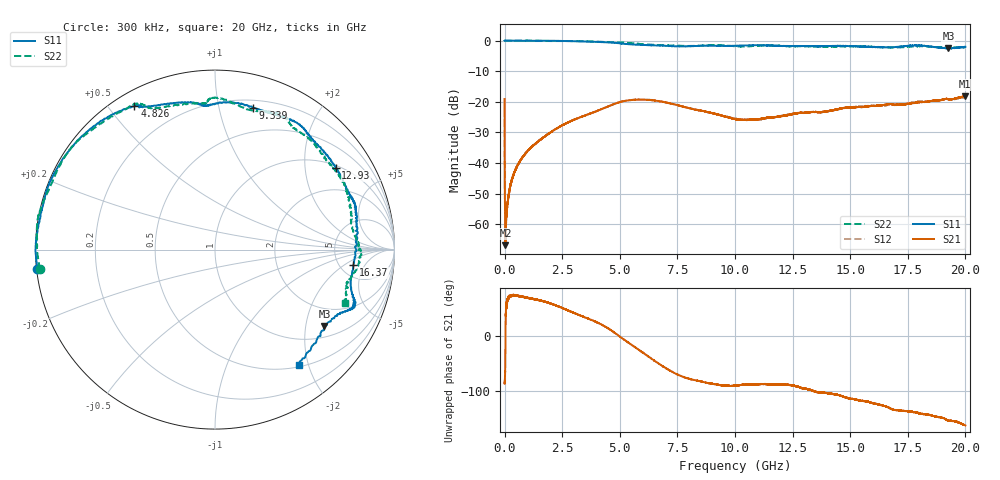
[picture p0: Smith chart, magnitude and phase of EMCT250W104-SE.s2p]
!EMCT250W104
!Johanson Technology Inc.
!www.johansontechnology.com
!Test Board Conditions:
!Substrate Type  RO4350B
!Substrate Thickness  10 mil
!Substrate Dk  3.66
!TL Type: GCPW
!TL Trace Width  22 mil
!TL Gap  14 mil
!PART MODE SINGLE ENDED (AKA BYPASS)
!DUT TOPOLOGY	SERIES-SHUNT
# MHz S  dB  R 50
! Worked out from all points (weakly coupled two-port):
!   20001 points, 300 kHz to 20 GHz, reference 50 ohm
!   highest |S21| = -18.23 dB at 20 GHz (marker M1); lowest = -66.9 dB at 38.3 MHz (marker M2)
!   lowest |S11| = -2.6 dB at 19.26 GHz (marker M3), VSWR 6.80, Z = 67 - j128 ohm
!   |S11| at or under -10 dB: nowhere
!   |S22| runs from -2.4 to 0.0 dB; largest |S21 - S12| = 0.0051
!   S11 on the Smith chart (normalised r, x): 300 kHz: 0.00, -0.05; 4.826 GHz: 0.06, +0.58; 9.339 GHz: 0.27, +1.27; 12.93 GHz: 1.08, +2.89; 16.37 GHz: 6.66, -2.86; 20 GHz: 0.53, -1.84
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0.3  -0.03 -173.8  -19.10 -82.9  -19.04 -82.9  -0.15 -173.6
38.299  -0.01 179.6  -66.93 -5.6  -66.68 -5.7  -0.07 179.7
111.298  -0.01 178.6  -54.55 61.7  -54.35 62.5  -0.08 179.0
209.297  -0.01 177.7  -48.79 70.6  -48.95 72.4  -0.07 177.8
356.295  -0.04 176.0  -44.52 73.7  -44.41 73.3  -0.05 176.2
871.287  -0.07 170.4  -37.16 69.7  -37.34 69.8  0.03 170.2
2002.27  -0.06 156.8  -29.96 58.3  -29.87 58.3  -0.16 157.8
3334.25  -0.28 136.8  -24.89 35.9  -24.93 35.9  -0.18 143.0
4826.228  -0.76 119.3  -20.52 4.1  -20.55 4.0  -0.60 125.1
6667.2  -1.61 99.3  -19.76 -49.7  -19.72 -50.2  -1.45 110.7
7881.182  -1.88 92.7  -21.85 -76.2  -21.82 -75.9  -1.74 95.4
9339.16  -1.75 75.0  -24.32 -89.1  -24.34 -88.6  -1.49 87.9
10000.15  -1.72 66.9  -25.64 -90.3  -25.48 -90.3  -1.85 79.7
12928.11  -1.81 34.1  -23.64 -95.1  -23.62 -95.7  -1.85 50.8
13334.1  -1.85 27.7  -23.36 -99.0  -23.33 -99.2  -1.90 45.3
15178.07  -1.82 13.0  -21.84 -114.8  -21.68 -114.4  -1.86 25.7
16365.06  -2.21 -6.3  -21.09 -125.9  -21.27 -126.8  -2.12 14.5
16667.05  -2.22 -11.4  -20.75 -130.1  -21.01 -129.3  -2.22 12.2
17905.03  -1.61 -22.7  -20.25 -139.2  -20.01 -139.4  -1.87 -1.7
19264.01  -2.57 -34.9  -19.19 -153.8  -19.28 -154.7  -2.42 -14.1
19999  -2.01 -54.0  -18.23 -162.4  -18.44 -160.8  -2.14 -22.6
20000  -2.01 -54.2  -18.26 -162.4  -18.44 -160.7  -2.13 -22.5
